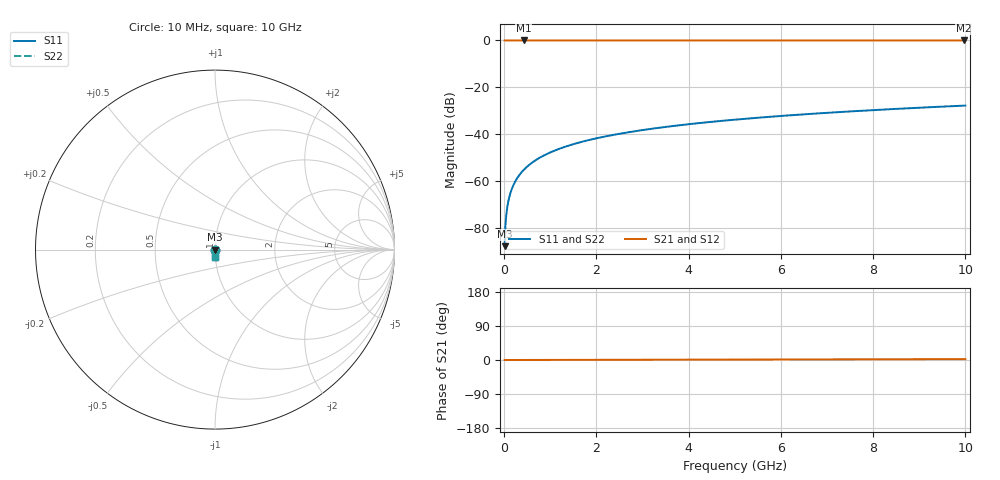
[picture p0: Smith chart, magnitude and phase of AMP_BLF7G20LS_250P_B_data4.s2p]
! AWR Design Environment (6079) Fri Apr 26 14:20:18 2013
! Simulator: Linear circuit simulator
! Ports: 2, Freqs: 1001
# GHz S MA R 50
!Freq  MagS11  AngS11  MagS21  AngS21  MagS12  AngS12  MagS22  AngS22
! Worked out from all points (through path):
!   1000 points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, 10 MHz to 10 GHz, reference 50 ohm
!   highest |S21| = 0.00 dB at 420 MHz (marker M1); lowest = 0.0 dB at 9.96 GHz (marker M2)
!   lowest |S11| = -87.8 dB at 10 MHz (marker M3), VSWR 1.00, Z = 50 - j0.00408 ohm
!   |S11| at or under -10 dB: start of sweep to end of sweep
!   |S22| runs from -87.8 to -27.8 dB; largest |S21 - S12| = 0
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0.01  4.084e-05 -90.0  1 0.0  1 0.0  4.084e-05 -90.0
0.04  0.0001634 -90.0  1 0.0  1 0.0  0.0001634 -90.0
0.1  0.0004084 -90.0  1 0.0  1 0.0  0.0004084 -90.0
0.13  0.0005309 -90.0  1 0.0  1 0.0  0.0005309 -90.0
0.16  0.0006534 -90.0  1 0.0  1 0.0  0.0006534 -90.0
0.21  0.0008576 -90.0  1 0.0  1 0.0  0.0008576 -90.0
0.27  0.001103 -89.9  1 0.1  1 0.1  0.001103 -89.9
0.34  0.001389 -89.9  1 0.1  1 0.1  0.001389 -89.9
0.42  0.001715 -89.9  1 0.1  1 0.1  0.001715 -89.9
0.52  0.002124 -89.9  1 0.1  1 0.1  0.002124 -89.9
0.63  0.002573 -89.9  1 0.1  1 0.1  0.002573 -89.9
0.91  0.003717 -89.8  1 0.2  1 0.2  0.003717 -89.8
1.26  0.005146 -89.7  1 0.3  1 0.3  0.005146 -89.7
1.68  0.006861 -89.6  1 0.4  1 0.4  0.006861 -89.6
2.41  0.009842 -89.4  1 0.6  1 0.6  0.009842 -89.4
3.34  0.01364 -89.2  0.9999 0.8  0.9999 0.8  0.01364 -89.2
4.12  0.01682 -89.0  0.9999 1.0  0.9999 1.0  0.01682 -89.0
5.01  0.02046 -88.8  0.9998 1.2  0.9998 1.2  0.02046 -88.8
6.67  0.02723 -88.4  0.9996 1.6  0.9996 1.6  0.02723 -88.4
8.34  0.03404 -88.0  0.9994 2.0  0.9994 2.0  0.03404 -88.0
9.96  0.04064 -87.7  0.9992 2.3  0.9992 2.3  0.04064 -87.7
10  0.04081 -87.7  0.9992 2.3  0.9992 2.3  0.04081 -87.7
